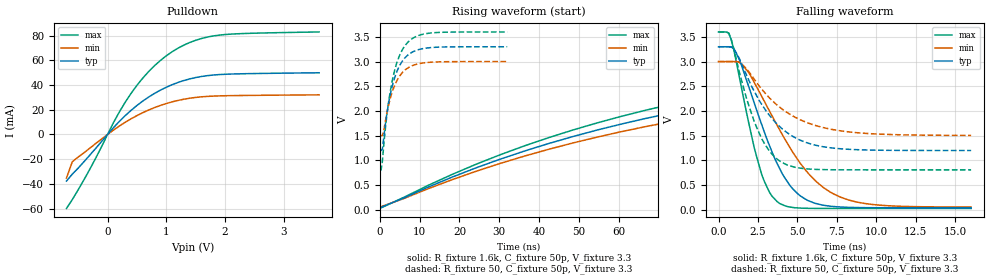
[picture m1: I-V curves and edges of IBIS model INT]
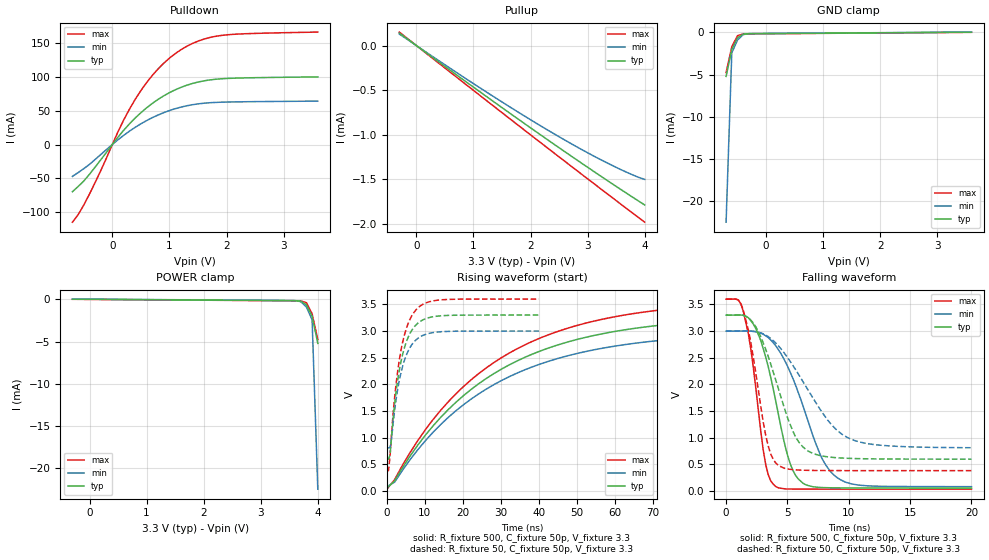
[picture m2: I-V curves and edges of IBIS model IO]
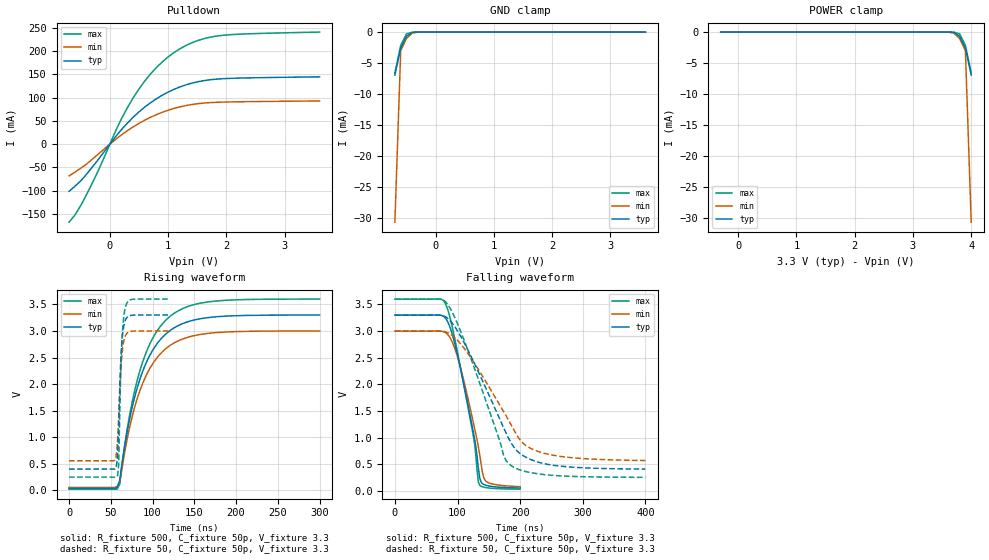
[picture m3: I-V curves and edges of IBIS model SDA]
[IBIS Ver]   3.2
[Comment Char]   |_char
| VDD Nom: 3.3v, Min: 3v, Max: 3.6v
[File name]   pca9674_3_3v.ibs
[File Rev]   1
[Date]   08-25-2008
[Source]
[Notes]
[Disclaimer]
(C) Copyright 2007 NXP Semiconductors
All rights reserved
NXP Semiconductors (NXP) does not warrant that this model and any other
accompanying information (Model) accurately or fully represents the
operating characteristics and specifications of the semiconductor
products to which the Model relates.  Moreover, the Model is furnished
on an "as is" and with "all faults" basis, and without support or
warranty of any kind.  NXP disclaims all warranties, whether expressed
or implied or statutory, including without limitation all implied
warranties of non-infringement, merchantability and fitness for any
purpose, and those arising from a course of dealing or usage of trade.
NXP does not convey any license under its or any third party's patents,
copyrights or other intellectual property or proprietary rights.
You and your company assume any and all risks and liability arising out
of the application or use of the Model.
In no event shall NXP be liable for any direct, indirect, special,
consequential or incidental damages, however caused, whether in
warranty, contract or tort (including negligence), strict liability or
other legal theory, including, without limitation, for lost profits,
business interruption, or corruption or loss of data or information,
arising out of or in connection with the use of or the inability to use
the Model, even if NXP has been advised of the possibility of such
damages.
NXP provides the Model as a courtesy to our customers. You and your
company shall not distribute, convey, sell, or give the Model to anyone
else without receiving prior written permission from NXP.
NXP reserves the right to make changes without notice to the Model to
improve reliability, function, or design.
Please be aware that your receipt and subsequent use of the Model shall
serve as acceptance of these terms and conditions.  If you do not
accept these terms, return or destroy the Model immediately.
[Copyright]
2008
| SO16 package
[Component]   PCA9674D
Si_location Pin
Timing_location Pin
[Manufacturer]   NXP Semiconductors
[Package]
R_pkg   1.75E-01   1.28E-01   2.11E-01
L_pkg   5.03E-09   3.94E-09   6.26E-09
C_pkg   0.794p   0.715p   0.869p
[Pin] signal_name   model_name   R_pin   L_pin   C_pin
1   AD0   ADDR   1.99E-01  6.26E-09  8.22E-13
2   AD1   ADDR   2.11E-01  5.46E-09  8.69E-13
3   AD2   ADDR   1.56E-01  4.44E-09  7.60E-13
4   P0   IO   1.28E-01  3.94E-09  7.17E-13
5   P1   IO   1.28E-01  3.94E-09  7.15E-13
6   P2   IO   1.56E-01  4.44E-09  7.60E-13
7   P3   IO   2.11E-01  5.46E-09  8.69E-13
8   VSS   GND   1.99E-01  6.26E-09  8.43E-13
9   P4   IO   1.99E-01  6.26E-09  8.43E-13
10   P5   IO   2.11E-01  5.46E-09  8.69E-13
11   P6   IO   1.56E-01  4.44E-09  7.60E-13
12   P7   IO   1.28E-01  3.94E-09  7.17E-13
13   INTb   INT   1.28E-01  3.94E-09  7.15E-13
14   SCL   SCL   1.56E-01  4.44E-09  7.60E-13
15   SDA   SDA   2.11E-01  5.46E-09  8.69E-13
16   VDD   POWER   1.99E-01  6.26E-09  8.43E-13
| TSSOP16 package
[Component]   PCA9674PW
Si_location Pin
Timing_location Pin
[Manufacturer]   NXP Semiconductors
[Package]
R_pkg   3.95E-02   3.52E-02   4.56E-02
L_pkg   1.94n   1.65n   2.40n
C_pkg   .446p   .335p   .771p
[Pin] signal_name   model_name   R_pin   L_pin   C_pin
1   AD0   ADDR   3.52E-02  2.40E-09  4.36E-13
2   AD1   ADDR   3.70E-02  1.93E-09  4.38E-13
3   AD2   ADDR   4.56E-02  1.76E-09  3.45E-13
4   P0   IO   4.00E-02  1.65E-09  3.35E-13
5   P1   IO   4.00E-02  1.65E-09  3.35E-13
6   P2   IO   4.56E-02  1.76E-09  3.45E-13
7   P3   IO   3.70E-02  1.93E-09  4.38E-13
8   VSS   GND   3.52E-02  2.40E-09  4.52E-13
9   P4   IO   3.52E-02  2.40E-09  4.52E-13
10   P5   IO   3.70E-02  1.93E-09  4.38E-13
11   P6   IO   4.56E-02  1.76E-09  3.45E-13
12   P7   IO   4.00E-02  1.65E-09  7.71E-13
13   INTb   ADDR   4.00E-02  1.65E-09  7.71E-13
14   SCL   SCL   4.56E-02  1.76E-09  3.45E-13
15   SDA   SDA   3.70E-02  1.93E-09  4.38E-13
16   VDD   POWER   3.52E-02  2.40E-09  4.52E-13
[Define Package Model]  HVQFN16
[Manufacturer]  ST-NXP Wireless
[OEM]  Unknown
[Description]  Full package model
|[Simulated] Chris Hunat
|[Approved] Wayne Nunn, Roger Real
[Number Of Pins]  16
[Pin Numbers]
|Pin Num   Terminal Name
1   | lead1:pin1
2   | lead2:pin2
3   | lead3:pin3
4   | lead4:pin4
5   | lead5:pin5
6   | lead6:pin6
7   | lead7:pin7
8   | lead8:pin8
9   | lead9:pin9
10   | lead10:pin10
11   | lead11:pin11
12   | lead12:pin12
13   | lead13:pin13
14   | lead14:pin14
15   | lead15:pin15
16   | lead16:pin16
[Model Data]
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[End Model Data]
[End Package Model]
| Models and submodels in the file (5): INT (Open_drain), IO (I/O), SDA (I/O_open_drain), SCL (Input), ADDR (Input)
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[Model]   INT
Model_type Open_drain
Vref=3.3
Vmeas=1.65
Rref=500
Cref=50p
C_comp   5.2p   5p   5.4p
[Temperature Range] 27   85   -40
[Voltage Range]   3.3   3   3.6
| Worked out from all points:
|   slope of the pulldown table from 0 to 0.495 V, typ, clamps not added: 21.3 ohm
|   falling waveform, R_fixture 1.6k, C_fixture 50p, V_fixture 3.3: 20-80 % time 2.36ns typ, 3.42ns min, 1.52ns max; typ from 3.3 V to 0.037 V
|   falling waveform, R_fixture 50, C_fixture 50p, V_fixture 3.3: 20-80 % time 2.54ns typ, 3.17ns min, 1.74ns max; typ from 3.3 V to 1.2 V
|   rising waveform, R_fixture 1.6k, C_fixture 50p, V_fixture 3.3: 20-80 % time 112ns typ, 113ns min, 112ns max; typ from 0.037 V to 3.3 V
|   rising waveform, R_fixture 50, C_fixture 50p, V_fixture 3.3: 20-80 % time 3.52ns typ, 3.52ns min, 3.51ns max; typ from 1.2 V to 3.3 V
[Pulldown]
-700mV    -37.76mA   -35.32mA   -59.97mA
-600mV    -32.14mA   -22.14mA   -52.74mA
-300mV    -16.65mA   -11.05mA   -27.99mA
100mV     5.453mA    3.495mA    9.476mA
300mV     15.19mA    9.813mA    26.06mA
600mV     27.02mA    17.6mA     45.64mA
800mV     33.23mA    21.72mA    55.68mA
1V        38.22mA    25.02mA    63.67mA
1.4V      44.97mA    29.32mA    74.46mA
1.8V      48.09mA    31.03mA    79.74mA
2.3V      49.12mA    31.53mA    81.67mA
3.6V      49.91mA    32.03mA    82.97mA
[Falling Waveform]
R_fixture=1.6k
C_fixture=50p
V_fixture=3.3
V_fixture_min=3
V_fixture_max=3.6
0s        3.3V       3V         3.6V
646.5ps   3.3V       3V         3.577V
1.131ns   3.163V     2.999V     2.987V
2.263ns   2.162V     2.578V     1.254V
2.747ns   1.712V     2.289V     700.3mV
3.232ns   1.293V     1.995V     347.3mV
3.879ns   828.2mV    1.614V     122.9mV
5.495ns   213.5mV    809.4mV    26.97mV
7.758ns   52.15mV    248.7mV    22.92mV
16ns      36.62mV    52.66mV    22.88mV
[Falling Waveform]
R_fixture=50
C_fixture=50p
V_fixture=3.3
V_fixture_min=3
V_fixture_max=3.6
0s        3.3V       3V         3.6V
646.5ps   3.3V       3V         3.578V
969.7ps   3.259V     3V         3.261V
1.455ns   2.962V     2.957V     2.624V
2.263ns   2.398V     2.643V     1.785V
2.747ns   2.128V     2.437V     1.43V
4.202ns   1.593V     1.997V     926.1mV
5.657ns   1.348V     1.756V     824.1mV
8.081ns   1.225V     1.581V     805.8mV
16ns      1.197V     1.503V     805mV
[Rising Waveform]
R_fixture=1.6k
C_fixture=50p
V_fixture=3.3
V_fixture_min=3
V_fixture_max=3.6
0s        36.62mV    51.97mV    22.88mV
30.3ns    1.024V     937.3mV    1.114V
48.48ns   1.48V      1.35V      1.613V
66.67ns   1.845V     1.68V      2.012V
84.85ns   2.137V     1.944V     2.331V
109.1ns   2.437V     2.216V     2.659V
163.6ns   2.859V     2.6V       3.12V
224.2ns   3.091V     2.81V      3.373V
303ns     3.221V     2.928V     3.514V
600ns     3.298V     2.998V     3.598V
[Rising Waveform]
R_fixture=50
C_fixture=50p
V_fixture=3.3
V_fixture_min=3
V_fixture_max=3.6
0s        1.197V     1.502V     805mV
323.2ps   1.197V     1.502V     805mV
646.5ps   1.233V     1.502V     987.4mV
1.293ns   1.667V     1.748V     1.569V
1.939ns   2.032V     2.025V     2.024V
3.232ns   2.539V     2.415V     2.659V
4.848ns   2.898V     2.691V     3.103V
6.788ns   3.113V     2.857V     3.37V
12.61ns   3.281V     2.986V     3.577V
32ns      3.3V       3V         3.6V
[Ramp]
R_load=1.6k
dV/dt_r   1.958E+0/1.851E-9   1.946E+0/2.033E-9   1.967E+0/1.628E-9
dV/dt_f   1.958E+0/1.637E-10   1.946E+0/2.065E-10   1.967E+0/7.359E-11
|[End   INT
| [End   IO
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[Model]   IO
Model_type I/O
Vinh=2.31
Vinl=0.99
Vref=3.3
Vmeas=1.65
Rref=500
Cref=50p
C_comp   7p   6.8p   7.2p
[Temperature Range] 27   85   -40
[Voltage Range]   3.3   3   3.6
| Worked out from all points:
|   slope of the pulldown table from 0 to 0.495 V, typ, clamps not added: 10.7 ohm
|   slope of the pullup table from 0 to 0.495 V, typ, clamps not added: 2.13 kohm
|   GND clamp passes 1 mA (typ) near -0.52 V on its own axis
|   falling waveform, R_fixture 500, C_fixture 50p, V_fixture 3.3: 20-80 % time 1.92ns typ, 2.86ns min, 1.18ns max; typ from 3.3 V to 0.059 V
|   falling waveform, R_fixture 50, C_fixture 50p, V_fixture 3.3: 20-80 % time 2.36ns typ, 3.75ns min, 1.38ns max; typ from 3.3 V to 0.6 V
|   rising waveform, R_fixture 500, C_fixture 50p, V_fixture 3.3: 20-80 % time 34.7ns typ, 34.9ns min, 34.6ns max; typ from 0.059 V to 3.3 V
|   rising waveform, R_fixture 50, C_fixture 50p, V_fixture 3.3: 20-80 % time 3.57ns typ, 3.59ns min, 3.56ns max; typ from 0.6 V to 3.3 V
[Pullup]
-300mV    140.2uA    129.3uA    150.8uA
1.1V      -512.3uA   -468.2uA   -552.5uA
2.3V      -1.056mA   -947uA     -1.149mA
2.8V      -1.277mA   -1.131mA   -1.395mA
3.3V      -1.493mA   -1.302mA   -1.64mA
3.7V      -1.662mA   -1.425mA   -1.835mA
4V        -1.787mA   -1.5mA     -1.98mA
[Pulldown]
-700mV    -69.7mA    -47.05mA   -114.6mA
-600mV    -61.98mA   -41.49mA   -103.5mA
-400mV    -43.82mA   -29.24mA   -72.96mA
-200mV    -22.2mA    -14.51mA   -37.9mA
100mV     11.05mA    7.118mA    19.12mA
400mV     39.11mA    25.38mA    66.64mA
700mV     60.68mA    39.63mA    102mA
900mV     71.84mA    47.03mA    119.9mA
1.1V      80.68mA    52.82mA    134.1mA
1.5V      92.18mA    59.98mA    152.6mA
1.9V      96.96mA    62.43mA    160.9mA
3.6V      99.8mA     64.04mA    165.9mA
[GND Clamp]
-700mV    -5.214mA   -22.45mA   -4.761mA
-600mV    -2.033mA   -2.422mA   -1.708mA
-500mV    -655.6uA   -909.6uA   -400.5uA
-400mV    -212.8uA   -276uA     -193uA
-200mV    -158.7uA   -141uA     -176.5uA
3.6V      13.62uA    27.33uA    109.1pA
[POWER Clamp]
-300mV    13.62uA    27.33uA    109.1pA
3.5V      -158.7uA   -141uA     -176.5uA
3.7V      -212.8uA   -276uA     -193uA
3.8V      -655.6uA   -909.6uA   -400.5uA
3.9V      -2.033mA   -2.422mA   -1.708mA
4V        -5.214mA   -22.45mA   -4.761mA
[Falling Waveform]
R_fixture=500
C_fixture=50p
V_fixture=3.3
V_fixture_min=3
V_fixture_max=3.6
0s        3.3V       3V         3.6V
1.414ns   3.296V     3.001V     3.361V
2.02ns    3.193V     2.999V     2.659V
3.232ns   2.511V     2.911V     495.3mV
4.04ns    1.695V     2.728V     86.12mV
5.051ns   638.1mV    2.321V     39.9mV
5.657ns   298.4mV    1.991V     38.06mV
7.677ns   68.69mV    681.9mV    36.84mV
9.091ns   61.17mV    246.7mV    36.7mV
20ns      58.61mV    83.38mV    36.65mV
[Falling Waveform]
R_fixture=50
C_fixture=50p
V_fixture=3.3
V_fixture_min=3
V_fixture_max=3.6
0s        3.3V       3V         3.6V
1.414ns   3.296V     3.001V     3.381V
2.02ns    3.204V     2.999V     2.782V
3.232ns   2.656V     2.923V     1.042V
4.242ns   1.936V     2.728V     485.7mV
5.455ns   1.12V      2.353V     402.8mV
6.263ns   829.5mV    2.054V     392.3mV
8.283ns   642.6mV    1.33V      385.4mV
9.899ns   615.3mV    1.004V     384.5mV
20ns      599.6mV    813.4mV    384.2mV
[Rising Waveform]
R_fixture=500
C_fixture=50p
V_fixture=3.3
V_fixture_min=3
V_fixture_max=3.6
0s        58.6mV     83.02mV    36.65mV
2.02ns    194.9mV    169.6mV    217.3mV
6.061ns   654.8mV    587mV      720.5mV
12.12ns   1.222V     1.102V     1.34V
22.22ns   1.909V     1.728V     2.09V
36.36ns   2.509V     2.275V     2.743V
52.53ns   2.886V     2.619V     3.152V
70.71ns   3.1V       2.816V     3.384V
96.97ns   3.23V      2.935V     3.525V
200ns     3.299V     2.999V     3.599V
[Rising Waveform]
R_fixture=50
C_fixture=50p
V_fixture=3.3
V_fixture_min=3
V_fixture_max=3.6
0s        599.5mV    809.9mV    384.2mV
404ps     599.5mV    809.9mV    384.5mV
808.1ps   675.1mV    817mV      657.9mV
1.212ns   1.027V     987.2mV    1.086V
2.02ns    1.637V     1.52V      1.763V
3.636ns   2.409V     2.202V     2.621V
5.253ns   2.827V     2.576V     3.081V
7.677ns   3.118V     2.836V     3.401V
14.14ns   3.286V     2.987V     3.584V
40ns      3.3V       3V         3.6V
[Ramp]
R_load=500
dV/dt_r   4.388E-2/1.281E-9   3.871E-2/1.430E-9   4.901E-2/1.040E-9
dV/dt_f   1.944E+0/5.484E-10   1.746E+0/9.304E-10   2.138E+0/2.734E-10
|[End   IO
| [End   SDA
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[Model]   SDA
Model_type I/O_open_drain
Vinh=2.31
Vinl=0.99
Vref=3.3
Vmeas=1.65
Rref=1k
Cref=50p
C_comp   6p   5.8p   6.2p
[Temperature Range] 27   85   -40
[Voltage Range]   3.3   3   3.6
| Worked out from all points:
|   slope of the pulldown table from 0 to 0.495 V, typ, clamps not added: 7.2 ohm
|   GND clamp passes 1 mA (typ) near -0.52 V on its own axis
|   falling waveform, R_fixture 500, C_fixture 50p, V_fixture 3.3: 20-80 % time 32.7ns typ, 33.2ns min, 33.5ns max; typ from 3.3 V to 0.051 V
|   falling waveform, R_fixture 50, C_fixture 50p, V_fixture 3.3: 20-80 % time 68.4ns typ, 73.8ns min, 60.6ns max; typ from 3.3 V to 0.407 V
|   rising waveform, R_fixture 500, C_fixture 50p, V_fixture 3.3: 20-80 % time 35.4ns typ, 35.5ns min, 35.3ns max; typ from 0.039 V to 3.3 V
|   rising waveform, R_fixture 50, C_fixture 50p, V_fixture 3.3: 20-80 % time 4.02ns typ, 4.65ns min, 3.77ns max; typ from 0.401 V to 3.3 V
[Pulldown]
-700mV    -101.5mA   -68.23mA   -167.9mA
-600mV    -90.64mA   -60.36mA   -152.5mA
-400mV    -64.71mA   -42.87mA   -108.7mA
-200mV    -33.19mA   -21.54mA   -57.19mA
200mV     31.35mA    19.98mA    54.76mA
400mV     57.83mA    37.18mA    99.59mA
700mV     89.28mA    57.92mA    151.2mA
1V        112.1mA    73.01mA    187.6mA
1.4V      131.1mA    85.2mA     217.8mA
1.8V      139.6mA    89.94mA    232mA
2.3V      142.4mA    91.39mA    237.1mA
3.6V      144.9mA    92.99mA    241.2mA
[GND Clamp]
-700mV    -6.935mA   -30.66mA   -6.593mA
-600mV    -2.591mA   -2.99mA    -2.148mA
-500mV    -653.7uA   -1.019mA   -278.6uA
-400mV    -54.45uA   -160.3uA   -7.607uA
-200mV    -25.65nA   -197.3nA   -667.7pA
3.6V      201.4pA    372.1pA    187.3pA
[POWER Clamp]
-300mV    201.4pA    372.1pA    187.3pA
3.5V      -25.65nA   -197.3nA   -667.7pA
3.7V      -54.45uA   -160.3uA   -7.607uA
3.8V      -653.7uA   -1.019mA   -278.6uA
3.9V      -2.591mA   -2.99mA    -2.148mA
4V        -6.935mA   -30.66mA   -6.593mA
[Falling Waveform]
R_fixture=500
C_fixture=50p
V_fixture=3.3
V_fixture_min=3
V_fixture_max=3.6
0s        3.3V       3V         3.6V
78.79ns   3.268V     2.984V     3.553V
88.89ns   3.042V     2.858V     3.215V
103ns     2.387V     2.39V      2.417V
125.3ns   1.101V     1.282V     1.034V
133.3ns   426.1mV    826.3mV    164.6mV
135.4ns   250.7mV    681.8mV    104.8mV
141.4ns   122.1mV    264.8mV    70.15mV
145.5ns   104.2mV    177.8mV    60.03mV
200ns     51.46mV    77.03mV    30.61mV
[Falling Waveform]
R_fixture=50
C_fixture=50p
V_fixture=3.3
V_fixture_min=3
V_fixture_max=3.6
0s        3.3V       3V         3.6V
72.73ns   3.298V     2.999V     3.599V
84.85ns   3.236V     2.968V     3.493V
117.2ns   2.631V     2.57V      2.621V
165.7ns   1.395V     1.647V     998.2mV
173.7ns   1.183V     1.485V     656.7mV
185.9ns   894.7mV    1.234V     471.4mV
206.1ns   650.9mV    879.2mV    369.6mV
238.4ns   510.1mV    704.7mV    304.2mV
400ns     407mV      568.6mV    252.9mV
[Rising Waveform]
R_fixture=500
C_fixture=50p
V_fixture=3.3
V_fixture_min=3
V_fixture_max=3.6
0s        39.15mV    56.18mV    24.11mV
57.58ns   50.17mV    74.27mV    23.92mV
60.61ns   185.4mV    154.2mV    117.1mV
66.67ns   839.7mV    719.9mV    851.4mV
75.76ns   1.576V     1.401V     1.675V
87.88ns   2.228V     2.004V     2.405V
103ns     2.708V     2.45V      2.941V
124.2ns   3.043V     2.76V      3.314V
172.7ns   3.262V     2.964V     3.558V
300ns     3.3V       3V         3.6V
[Rising Waveform]
R_fixture=50
C_fixture=50p
V_fixture=3.3
V_fixture_min=3
V_fixture_max=3.6
0s        401.2mV    558.1mV    250.6mV
53.33ns   401.2mV    558mV      250.6mV
56.97ns   478.9mV    709.5mV    250.6mV
58.18ns   677.9mV    958mV      284.5mV
59.39ns   1.179V     1.364V     476.7mV
61.82ns   2.406V     2.209V     2.2V
63.03ns   2.746V     2.501V     2.727V
65.45ns   3.086V     2.806V     3.263V
67.88ns   3.218V     2.925V     3.471V
120ns     3.3V       3V         3.6V
[Ramp]
R_load=500
dV/dt_r   1.957E+0/1.366E-9   1.943E+0/1.981E-9   1.967E+0/8.995E-10
dV/dt_f   1.956E+0/3.194E-8   1.942E+0/3.578E-8   1.967E+0/2.977E-8
|[End   SDA
| [End   SCL
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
